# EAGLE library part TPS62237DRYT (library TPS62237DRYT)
Texas Instruments, TPS62237DRYT Step-Down Switching Regulator 500mA, 6-Pin SON Source: Datasheet
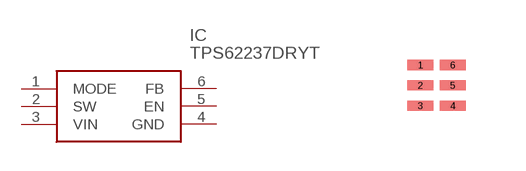
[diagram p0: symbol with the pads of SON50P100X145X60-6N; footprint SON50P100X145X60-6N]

Designator prefix IC

## TPS62237DRYT (Arrow_Part_Number: TPS62237DRYT; Arrow_Price/Stock: https://www.arrow.com/en/products/tps62237dryt/texas-instruments; Description: Texas Instruments, TPS62237DRYT Step-Down Switching Regulator 500mA, 6-Pin SON; Height: mm; Manufacturer_Name: Texas Instruments; Manufacturer_Part_Number: TPS62237DRYT; RS_Part_Number: 8256977P; RS_Price/Stock: http://uk.rs-online.com/web/p/products/8256977P)  [SON50P100X145X60-6N]
1  MODE
2  SW
3  VIN
4  GND
5  EN
6  FB

## Footprint SON50P100X145X60-6N (pad centres in mm)
SON50P100X145X60-6N
smd 0.66 x 0.254: 1 -0.406,0.508; 2 -0.406,0; 3 -0.406,-0.508; 4 0.406,-0.508; 5 0.406,0; 6 0.406,0.508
